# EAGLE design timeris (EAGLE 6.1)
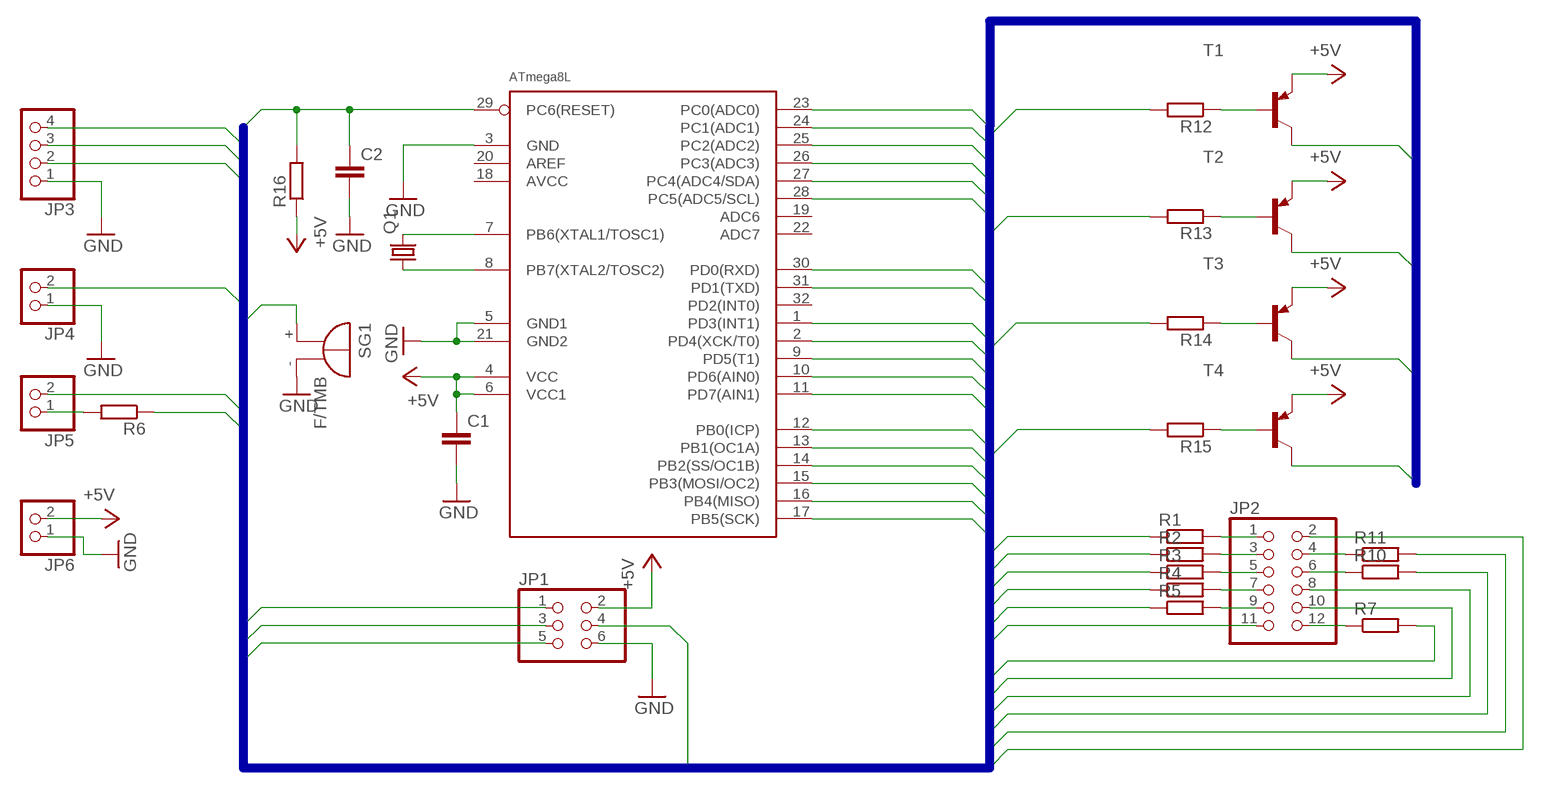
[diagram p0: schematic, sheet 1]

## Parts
C1  C-EUC1206  [C1206]
C2  C-EUC1206  [C1206]
JP1  PINHD-2X3  [2X03]
JP2  PINHD-2X6  [2X06]
JP3  PINHD-1X4  [1X04]
JP4  PINHD-1X2  [1X02]
JP5  PINHD-1X2  [1X02]
JP6  PINHD-1X2  [1X02]
Q1  CRYSTALHC49U-V  [HC49U-V]
R1  R-EU_M1206  [M1206]
R2  R-EU_M1206  [M1206]
R3  R-EU_M1206  [M1206]
R4  R-EU_M1206  [M1206]
R5  R-EU_M1206  [M1206]
R6  R-EU_M1206  [M1206]
R7  R-EU_M1206  [M1206]
R10  R-EU_M1206  [M1206]
R11  R-EU_M1206  [M1206]
R12  R-EU_M1206  [M1206]
R13  R-EU_M1206  [M1206]
R14  R-EU_M1206  [M1206]
R15  R-EU_M1206  [M1206]
R16  R-EU_M1206  [M1206]
SG1  F/TMB  [F/TMB]
T1  BC558A-PNP-TO92-EBC  [TO92-EBC]
T2  BC558A-PNP-TO92-EBC  [TO92-EBC]
T3  BC558A-PNP-TO92-EBC  [TO92-EBC]
T4  BC558A-PNP-TO92-EBC  [TO92-EBC]
U$1  ATMEGA8L  [ATMEGA8L]

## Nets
+5V: C1.1 JP1.2 JP6.2 R16.1 T1.E T2.E T3.E T4.E U$1.4(VCC) U$1.6(VCC1)
BUZZER: SG1.+ U$1.2(PD4(XCK/T0))
CA_1: JP2.2 T1.C
CA_2: JP2.8 T2.C
CA_3: JP2.10 T3.C
CA_4: JP2.11 T4.C
CA_B1: JP1.4 R12.2 U$1.15(PB3(MOSI/OC2))
CA_B2: R13.2 U$1.13(PB1(OC1A))
CA_B3: R14.2 U$1.14(PB2(SS/OC1B))
CA_B4: R15.2 U$1.12(PB0(ICP))
GND: C1.2 C2.2 JP1.6 JP3.1 JP4.1 JP6.1 SG1.- U$1.3(GND) U$1.5(GND1) U$1.21(GND2)
LED1_G: R6.1 U$1.10(PD6(AIN0))
LED1_R: JP5.2 U$1.9(PD5(T1))
N$1: JP2.1 R1.2
N$2: JP2.3 R2.2
N$3: JP2.5 R3.2
N$4: JP2.7 R4.2
N$5: JP2.9 R5.2
N$7: JP2.12 R7.1
N$10: JP2.6 R10.1
N$11: JP2.4 R11.1
N$12: R13.1 T2.B
N$13: R12.1 T1.B
N$14: R14.1 T3.B
N$15: R15.1 T4.B
N$40: Q1.2 U$1.7(PB6(XTAL1/TOSC1))
N$41: Q1.1 U$1.8(PB7(XTAL2/TOSC2))
N$42: JP5.1 R6.2
OUT: JP4.2 U$1.11(PD7(AIN1))
RST: C2.1 JP1.5 R16.2 U$1.29(PC6(RESET))
SEG_A: R11.2 U$1.28(PC5(ADC5/SCL))
SEG_B: JP1.1 R7.2 U$1.16(PB4(MISO))
SEG_C: R4.1 U$1.23(PC0(ADC0))
SEG_D: R2.1 U$1.25(PC2(ADC2))
SEG_DP: R3.1 U$1.24(PC1(ADC1))
SEG_E: R1.1 U$1.26(PC3(ADC3))
SEG_F: R10.2 U$1.27(PC4(ADC4/SDA))
SEG_G: JP1.3 R5.1 U$1.17(PB5(SCK))
SW_DOWN: JP3.2 U$1.30(PD0(RXD))
SW_START: JP3.4 U$1.1(PD3(INT1))
SW_UP: JP3.3 U$1.31(PD1(TXD))
Unconnected: U$1.18(AVCC) U$1.19(ADC6) U$1.20(AREF) U$1.22(ADC7) U$1.32(PD2(INT0))

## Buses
B$1
B$2

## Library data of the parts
C1 C2 = rcl:C-EU: CAPACITOR, European symbol
JP1 = pinhead:PINHD-2X3: PIN HEADER
JP2 = pinhead:PINHD-2X6: PIN HEADER
JP3 = pinhead:PINHD-1X4: PIN HEADER
JP4-JP6 = pinhead:PINHD-1X2: PIN HEADER
Q1 = crystal:CRYSTAL: CRYSTAL; OC_FARNELL: 1666969; OC_NEWARK: unknown
R1-R7 R10-R16 = rcl:R-EU_: RESISTOR, European symbol
SG1 = buzzer:F/TMB: BUZZER; OC_FARNELL: unknown; OC_NEWARK: unknown
T1-T4 = transistor:*-PNP-: PNP Transistror
U$1 = atmega8l:ATMEGA8L

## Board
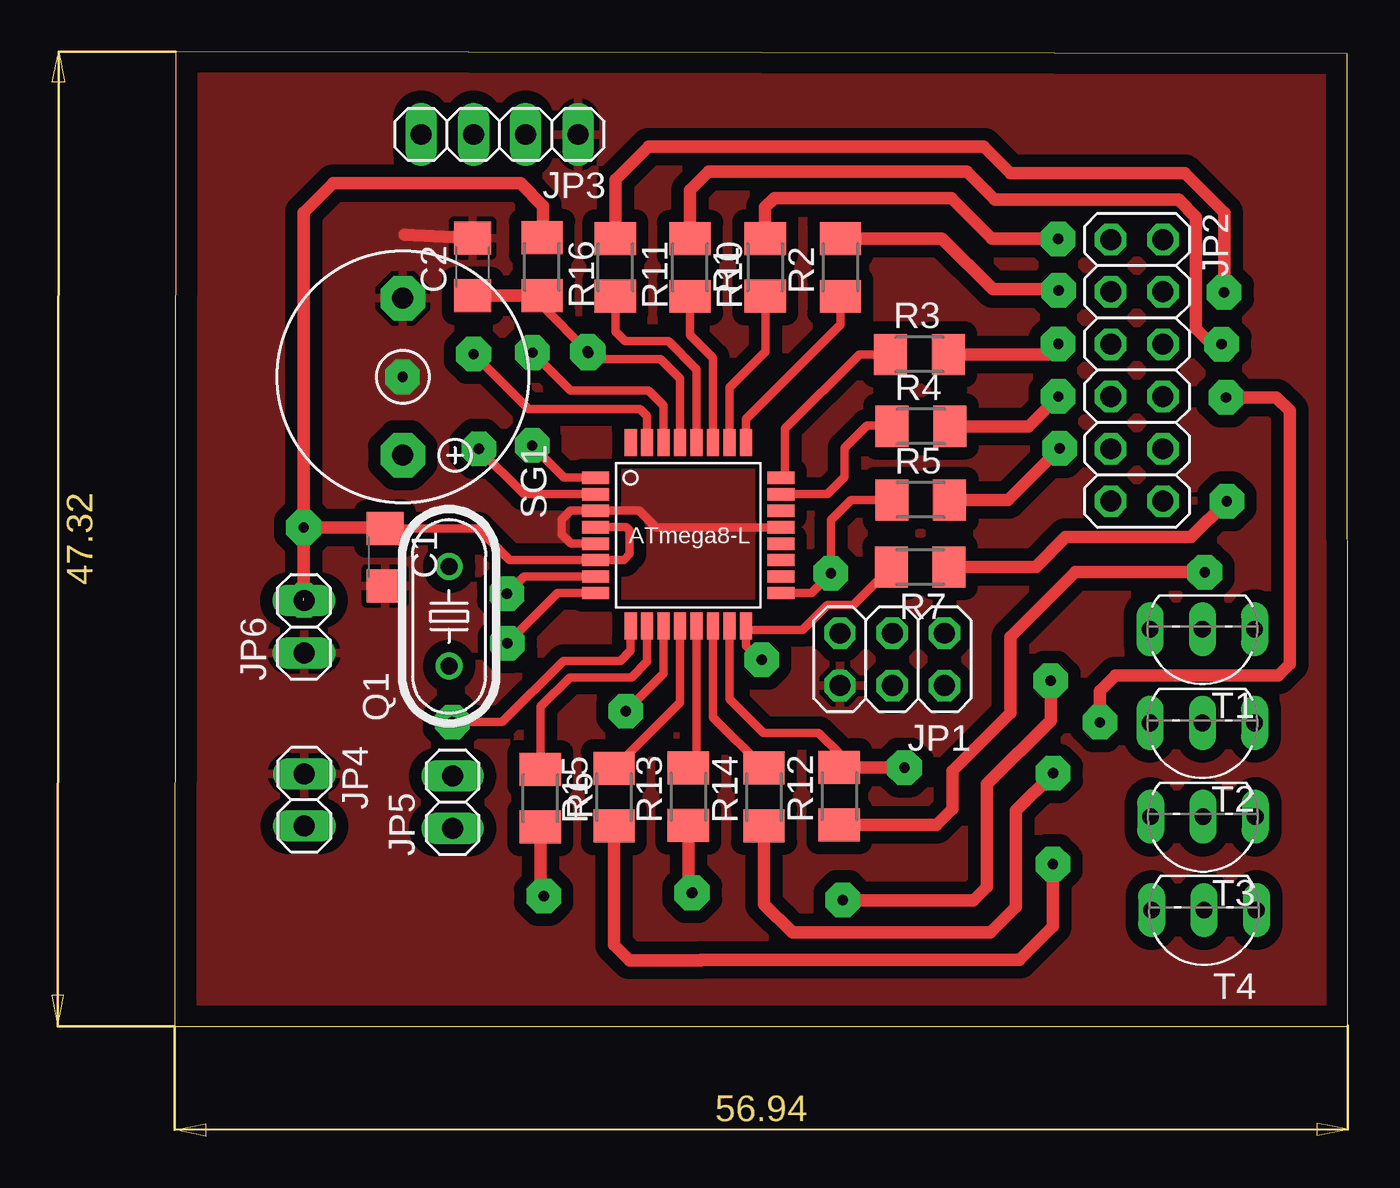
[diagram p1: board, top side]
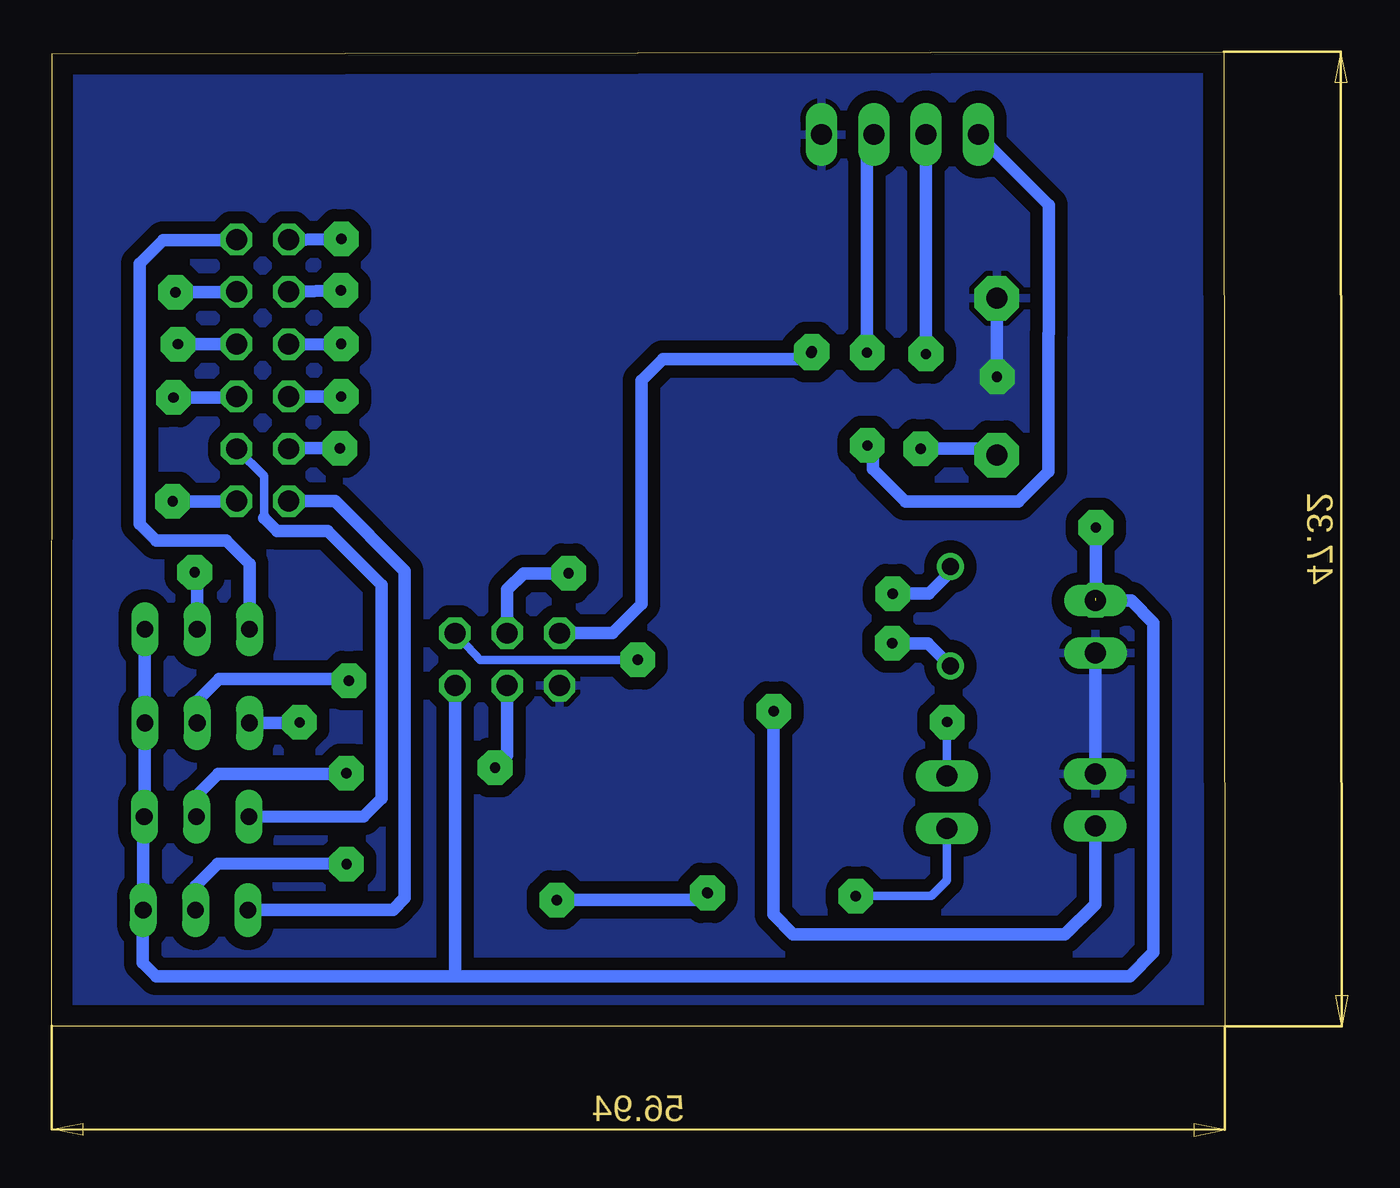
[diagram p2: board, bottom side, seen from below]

Size 62.93 x 52.65 mm. Coordinates in mm from the lower left corner, seen from the top.
Outline: 5.98,5.32 62.93,5.34 62.9,52.54 6.03,52.64 5.98,5.32
Copper layers (1*16): Top 0.035mm / dielectric 1.5mm / Bottom 0.035mm
Design rules: minimum track width 10mil, minimum drill 24mil, track to track 8mil, track to pad 8mil, pad to pad 8mil, via to via 8mil, smd to smd 8mil, copper to edge 40mil, drill to drill 8mil, minimum pad ring 10mil, minimum via ring 8mil, stop-mask expansion 4mil, vias tented up to drill 0mil, thermal gap 10mil

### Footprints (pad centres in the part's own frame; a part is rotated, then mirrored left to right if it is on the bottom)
C1206 = smd 1.6 x 1.8: 1 -1.4,0; 2 1.4,0
2X03 = drill 1.016 octagon: 1 -2.54,-1.27; 2 -2.54,1.27; 3 0,-1.27; 4 0,1.27; 5 2.54,-1.27; 6 2.54,1.27
2X06 = drill 1.016 octagon: 1 -6.35,-1.27; 2 -6.35,1.27; 3 -3.81,-1.27; 4 -3.81,1.27; 5 -1.27,-1.27; 6 -1.27,1.27; 7 1.27,-1.27; 8 1.27,1.27; 9 3.81,-1.27; 10 3.81,1.27; 11 6.35,-1.27; 12 6.35,1.27
1X04 = drill 1.016 long: 1 -3.81,0; 2 -1.27,0; 3 1.27,0; 4 3.81,0
1X02 = drill 1.016 long: 1 -1.27,0; 2 1.27,0
HC49U-V = drill 0.813: 1 -2.413,0; 2 2.413,0
M1206 = smd 1.6 x 2: 1 -1.4,0; 2 1.4,0
F/TMB = drill 1.016 pad 2.159 octagon: + 3.81,0; - -3.81,0
TO92-EBC = drill 0.813 long: B 0,-1.27; C 2.54,-1.27; E -2.54,-1.27
ATMEGA8L = smd 1.3 x 0.6: 1 -4.6,2.6; 2 -4.6,1.8; 3 -4.6,1; 4 -4.6,0.2; 5 -4.6,-0.6; 6 -4.6,-1.4; 7 -4.6,-2.2; 8 -4.6,-3; 17 4.4,-3; 18 4.4,-2.2; 19 4.4,-1.4; 20 4.4,-0.6; 21 4.4,0.2; 22 4.4,1; 23 4.4,1.8; 24 4.4,2.6 | smd 0.6 x 1.3: 9 -2.9,-4.6; 10 -2.1,-4.6; 11 -1.3,-4.6; 12 -0.5,-4.6; 13 0.3,-4.6; 14 1.1,-4.6; 15 1.9,-4.6; 16 2.7,-4.6; 25 2.7,4.3; 26 1.9,4.3; 27 1.1,4.3; 28 0.3,4.3; 29 -0.5,4.3; 30 -1.3,4.3; 31 -2.1,4.3; 32 -2.9,4.3

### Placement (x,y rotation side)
C1  16.19,28.09 270 top
C2  20.45,42.19 90 top
JP1  40.81,23.14 180 top
JP2  52.68,37.17 270 top
JP3  21.75,48.62 180 top
JP4  12.27,16.32 270 top
JP5  19.47,16.21 90 top
JP6  12.26,24.72 90 top
Q1  19.3,25.23 90 top
R1  34.64,42.17 90 top
R2  38.29,42.16 90 top
R3  42.13,37.94 0 top
R4  42.2,34.45 0 top
R5  42.19,30.88 0 top
R6  23.73,16.4 270 top
R7  42.16,27.63 180 top
R10  30.99,42.16 270 top
R11  27.37,42.17 270 top
R12  38.24,16.5 90 top
R13  30.91,16.47 90 top
R14  34.58,16.46 90 top
R15  27.3,16.45 90 top
R16  23.81,42.2 270 top
SG1  17.05,36.86 270 top
T1  55.86,23.33 180 top
T2  55.86,18.78 180 top
T3  55.89,14.23 180 top
T4  55.94,9.7 180 top
U$1  31.01,29.36 0 top

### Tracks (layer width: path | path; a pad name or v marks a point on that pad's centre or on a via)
+5V  (via drill 0.5 pad 1.68)  (1 unrouted)
  Top 0.406: U$1.4 27.9,29.56 28.07,29.39 28.07,28.25 27.78,27.96 U$1.6 22.23,27.96 20.7,29.49 C1.1
  Top 0.61: JP6.2 v12.25,26 12.25,44.83 13.67,46.25 22.76,46.25 23.87,45.14 23.87,43.66 R16.1 | C1.1 16.14,29.54 v12.24,29.54
  Bottom 0.61: T1.E T2.E 58.4,15.53 T3.E 58.48,15.45 T4.E 58.5,10.95 58.5,8.4 57.86,7.76 43.45,7.76 | v12.25,26 10.53,26 9.44,24.91 9.44,8.92 10.6,7.76 43.45,7.76 | JP1.2 43.35,7.86 43.45,7.76 | v12.24,29.54 v12.23,29.53 12.23,26.12
BUZZER  (via drill 0.5 pad 1.68)
  Top 0.406: U$1.2 22.94,31.16 v20.74,33.36
  Bottom 0.406: 20.74,33.38 v20.74,33.36
  Bottom 0.61: 20.74,33.38 17.38,33.38 SG1.+
CA_1
  Bottom 0.61: T1.C 53.32,27.76 54.46,28.9 57.84,28.9 58.65,29.71 58.65,42.34 57.5,43.49 53.98,43.49 JP2.2
CA_2  (via drill 0.5 pad 1.68)
  Top 0.61: v50.89,20.08 50.89,21.6 51.65,22.36 59.54,22.36 60.1,22.92 60.1,35.21 59.46,35.85 v57.01,35.85
  Bottom 0.61: JP2.8 54,35.85 v57.01,35.85 | T2.C 50.92,20.05 v50.89,20.08
CA_3
  Bottom 0.406: 52.62,30.01 52.62,32.03 JP2.10
  Bottom 0.61: T3.C 47.79,15.51 46.9,16.4 46.9,26.74 49.53,29.37 51.98,29.37 52.62,30.01
CA_4
  Bottom 0.61: T4.C 46.36,10.98 45.78,11.56 45.78,27.44 49.16,30.82 JP2.11
CA_B1  (via drill 0.5 pad 1.68)
  Top 0.406: U$1.15 32.91,21.22 34.56,19.57 37.24,19.57 38.26,18.55 38.26,17.92 R12.2
  Top 0.61: v41.4,17.89 R12.2
  Bottom 0.61: JP1.4 40.81,18.48 v41.4,17.89
CA_B2
  Top 0.406: U$1.13 31.31,18.27 R13.2
CA_B3
  Top 0.406: U$1.14 32.11,20.33 R14.2
CA_B4
  Top 0.406: U$1.12 30.51,21.06 R15.2
GND  (via drill 0.5 pad 1.68)
  Top 0.406: U$1.5 25.21,28.76 24.77,29.2 24.77,29.93 25.2,30.36 U$1.3 28.52,30.36 29.34,29.54 35.39,29.54 U$1.21
  Top 0.61: 17.13,43.76 C2.2
  Bottom 0.61: JP4.1 JP6.1 | SG1.- 17.04,36.8
  other vias: 17.04,36.86
  pour Bottom (isolate 0.61): 6.87,52.08 62.38,52.08 62.38,6.08 6.87,6.08
  pour Top (isolate 0.61): 6.86,52.06 62.38,52.06 62.38,6.08 6.86,6.08
LED1_G
  Top 0.406: 23.84,17.91 R6.1 23.74,20.85 25.16,22.27 28.15,22.27 28.91,23.03 U$1.10
LED1_R  (via drill 0.5 pad 1.68)
  Top 0.406: U$1.9 28.11,23.56 27.62,23.07 24.85,23.07 21.88,20.1 v19.46,20.1
  Bottom 0.406: v19.46,20.1 JP5.2
N$1  (via drill 0.5 pad 1.68)
  Top 0.61: 48.76,43.55 v48.86,43.55 45.65,43.55 43.67,45.53 35.09,45.53 34.64,45.08 R1.2
  Bottom 0.61: JP2.1 51.39,43.5 v48.86,43.55
N$2  (via drill 0.5 pad 1.68)
  Top 0.61: 48.84,41.05 v48.88,41.05 48.83,41.1 45.69,41.1 43.23,43.56 R2.2
  Bottom 0.61: JP2.3 51.39,41 v48.88,41.05
N$3  (via drill 0.5 pad 1.68)
  Top 0.61: 48.73,38.45 v48.87,38.45 48.36,37.94 R3.2
  Bottom 0.61: JP2.5 51.39,38.42 v48.87,38.45
N$4  (via drill 0.5 pad 1.68)
  Top 0.61: 48.81,35.9 v48.87,35.9 47.42,34.45 R4.2
  Bottom 0.61: v48.87,35.9 JP2.7
N$5  (via drill 0.5 pad 1.68)
  Top 0.61: 48.92,33.39 v48.94,33.39 46.43,30.88 R5.2
  Bottom 0.61: JP2.9 51.31,33.39 v48.94,33.39
N$7  (via drill 0.5 pad 1.68)
  Top 0.61: 57.07,30.81 v57.05,30.81 55.31,29.07 49.21,29.07 47.77,27.63 R7.1
  Bottom 0.61: JP2.12 v57.05,30.81
N$10  (via drill 0.5 pad 1.68)
  Top 0.61: 56.9,38.46 56.82,38.46 v56.8,38.44 56.3,38.44 55.55,39.19 55.55,44.61 54.71,45.45 45.79,45.45 44.43,46.81 31.89,46.81 30.99,45.91 R10.1
  Bottom 0.61: v56.8,38.44 JP2.6
N$11  (via drill 0.5 pad 1.68)
  Top 0.61: 56.95,40.96 v56.92,40.96 v56.93,40.97 56.93,44.83 55.01,46.75 46.54,46.75 45.26,48.03 28.97,48.03 27.37,46.43 R11.1
  Bottom 0.61: JP2.4 53.97,40.96 v56.92,40.96
N$12  (via drill 0.5 pad 1.68)
  Top 0.61: R13.1 30.92,12.01 v31.11,11.82 | v48.5,22.11 48.5,20.18 45.41,17.09 45.41,12.1 44.74,11.43 38.44,11.43 v38.41,11.46
  Bottom 0.61: T2.B 55.86,21.11 54.78,22.19 48.59,22.2 v48.5,22.11 | v31.08,11.79 v31.11,11.82 31.47,11.46 v38.41,11.46
N$13  (via drill 0.5 pad 1.68)
  Top 0.61: 38.22,15.08 R12.1 42.96,15.1 43.74,15.88 43.74,17.73 46.55,20.54 46.55,24.22 49.7,27.37 v55.98,27.37 55.97,27.17
  Bottom 0.61: T1.B 55.86,27.25 v55.98,27.37
N$14  (via drill 0.5 pad 1.68)
  Top 0.61: R14.1 34.58,11.26 35.96,9.88 45.57,9.88 46.81,11.12 46.81,15.8 v48.62,17.61
  Bottom 0.61: T3.B 55.89,16.53 54.84,17.58 48.64,17.59 v48.62,17.61
N$15  (via drill 0.5 pad 1.68)
  Top 0.61: v48.61,13.2 48.61,10.17 46.99,8.55 31.53,8.55 31.52,8.54 28.05,8.54 27.3,9.29 R15.1
  Bottom 0.61: T4.B 55.94,12.15 54.87,13.22 48.64,13.23 v48.61,13.2
N$40  (via drill 0.5 pad 1.68)
  Top 0.406: U$1.7 22.93,27.16 v22.1,26.33
  Bottom 0.61: v22.1,26.33 20.35,26.33 19.17,27.51 Q1.2
N$41  (via drill 0.5 pad 1.68)
  Top 0.406: U$1.8 24.56,26.36 v22.13,23.93
  Bottom 0.61: Q1.1 20.4,23.92 22.09,23.92 22.1,23.93 v22.13,23.93
N$42  (via drill 0.5 pad 1.68)
  Top 0.61: R6.2 23.73,11.81 v23.89,11.65
  Bottom 0.406: JP5.1 19.47,12.41 20.23,11.65 v23.89,11.65
  Bottom 0.61: v23.89,11.65 23.89,11.59 23.86,11.56
OUT  (via drill 0.5 pad 1.68)
  Top 0.406: U$1.11 29.71,22.46 v27.88,20.63
  Bottom 0.406: v27.88,20.63 27.76,20.63 27.74,20.61
  Bottom 0.61: JP4.2 12.27,11.26 13.74,9.79 26.93,9.79 27.9,10.76 27.9,20.61 v27.88,20.63
RST  (via drill 0.5 pad 1.68)
  Top 0.406: v26.02,38.09 23.81,40.3 R16.2 | U$1.29 30.51,36.76 29.55,37.72 26.36,37.72 v26.06,38.02
  Top 0.61: C2.1 R16.2
  Bottom 0.406: v26.06,38.02 26.06,38.05 v26.02,38.09
  Bottom 0.61: JP1.5 35.71,24.41 34.3,25.82 34.3,36.68 33.26,37.72 26.36,37.72 v26.06,38.02
SEG_A
  Top 0.406: U$1.28 31.31,37.21 29.94,38.58 27.84,38.58 27.38,39.04 R11.2
SEG_B  (via drill 0.5 pad 1.68)
  Top 0.406: v34.47,23.12 33.71,23.8 U$1.16 33.9,24.57 36.45,24.57 37.67,25.79 38.92,25.79 R7.2
  Bottom 0.406: v34.47,23.12 42.14,23.12 JP1.1
SEG_C
  Top 0.406: U$1.23 37.66,31.16 38.49,31.99 38.49,33.4 39.57,34.48 40.77,34.48 R4.1
SEG_D
  Top 0.406: U$1.25 33.71,34.8 38.3,39.39 R2.1
SEG_DP
  Top 0.406: R3.1 39.21,37.94 35.61,34.34 35.61,32.16 U$1.24
SEG_E
  Top 0.406: U$1.26 32.91,36.33 34.65,38.07 R1.1
SEG_F
  Top 0.406: R10.2 30.99,38.88 32.11,37.76 U$1.27
SEG_G  (via drill 0.5 pad 1.68)
  Top 0.406: R5.1 38.8,30.87 37.83,29.9 v37.83,27.32 v37.83,27.31 36.88,26.36 U$1.17
  Bottom 0.61: JP1.3 40.81,26.53 40.03,27.31 v37.84,27.31 v37.83,27.32
SW_DOWN  (via drill 0.5 pad 1.68)
  Top 0.406: U$1.30 29.71,35.47 28.99,36.19 25.19,36.19 v23.35,38.03
  Bottom 0.406: v23.35,38.03 23.35,38.12
  Bottom 0.61: JP3.2 23.35,48.29 v23.35,38.03
SW_START  (via drill 0.5 pad 1.68)
  Top 0.406: U$1.1 24.89,31.96 v23.33,33.52
  Bottom 0.406: v23.33,33.52 23.27,33.52 23.23,33.56
  Bottom 0.61: JP3.4 14.51,45.19 14.51,38.97 14.55,38.93 14.55,32.26 16.01,30.8 21.49,30.8 23.06,32.37 23.06,33.57 v23.33,33.52
SW_UP  (via drill 0.5 pad 1.68)
  Top 0.406: U$1.31 28.91,34.96 28.57,35.3 23.15,35.3 v20.49,37.96
  Bottom 0.406: v20.49,37.96 20.49,38.15
  Bottom 0.61: JP3.3 v20.49,37.96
